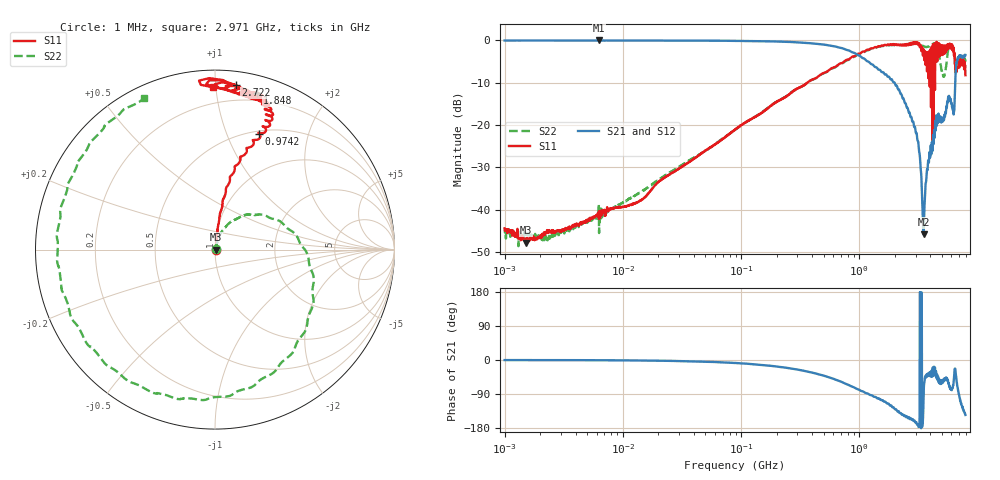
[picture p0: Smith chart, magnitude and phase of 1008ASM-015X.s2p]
!s-Parameter Generated by FASTRON Sdn. Bhd.
!FASTRON P/N : 1008ASM-015X
!Keysight Technologies: E5071C_MY46733604_B.14.02
!Date: Tue Nov 21 10:59:28 2023
!Version  :Rev00  Wed Nov 22 15:44:30 2023
!Data & Calibration Information:
!Freq  S11:SOLT2(ON)  S21:SOLT2(ON)  S12:SOLT2(ON)  S22:SOLT2(ON)
!PortZ  Port1:50+j0  Port2:50+j0
!When reading reference impedance value at option line is always used.
! Remarks : This data is being provided solely for informational purposes.
# Hz S dB R 50
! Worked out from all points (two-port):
!   1599 points, 1 MHz to 7.923 GHz, reference 50 ohm
!   highest |S21| = -0.03 dB at 6.301 MHz (marker M1); lowest = -45.8 dB at 3.508 GHz (marker M2)
!   |S21| within 3 dB of the highest: start of sweep to 920.1 MHz
!   lowest |S11| = -47.8 dB at 1.505 MHz (marker M3), VSWR 1.01, Z = 50.4 + j0.037 ohm
!   |S11| at or under -10 dB: start of sweep to 362.2 MHz; 3.950236 GHz to 3.957143 GHz (6.906 MHz wide, 0.175 % of centre); 4.141 GHz to 4.177 GHz (36.33 MHz wide, 0.873 % of centre)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
!   |S22| runs from -48.6 to -0.6 dB; largest |S21 - S12| = 0.012
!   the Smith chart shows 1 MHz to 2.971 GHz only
!   S11 on the Smith chart (normalised r, x): 1 MHz: 1.01, +0.00; 974.2 MHz: 0.53, +1.31; 1.848 GHz: 0.14, +1.29; 2.722 GHz: 0.09, +1.13; 2.971 GHz: 0.10, +0.98
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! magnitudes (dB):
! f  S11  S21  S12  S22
! 1 MHz  -44.4  0.0  0.0  -44.6
! 1.505 MHz  -47.8  0.0  0.0  -46.2
! 4.479 MHz  -42.9  0.0  -0.1  -43.5
! 6.301 MHz  -40.3  0.0  -0.1  -45.5
! 19.95 MHz  -33.4  -0.1  -0.1  -32.9
! 89.01 MHz  -21.1  -0.1  -0.1  -21.1
! 398.5 MHz  -9.3  -0.7  -0.7  -9.3
! 974.2 MHz  -3.2  -3.5  -3.5  -3.4
! 1.784 GHz  -1.1  -8.6  -8.6  -1.2
! 1.848 GHz  -0.9  -9.2  -9.2  -1.1
! 2.722 GHz  -0.7  -18.1  -18.1  -0.8
! 2.971 GHz  -0.9  -20.5  -20.5  -0.6
! 3.203 GHz  -0.8  -25.9  -25.9  -0.8
! 3.508 GHz  -2.1  -45.8  -45.9  -1.4
! 3.812 GHz  -2.8  -29.6  -29.6  -1.5
! 4.197 GHz  -3.8  -24.3  -24.3  -0.9
! 4.493 GHz  -3.5  -17.7  -17.7  -1.1
! 5.164 GHz  -3.1  -18.2  -18.2  -8.6
! 5.918 GHz  -0.9  -14.4  -14.4  -0.9
! 6.265 GHz  -2.7  -16.7  -16.6  -2.0
! 6.882 GHz  -4.6  -4.3  -4.3  -5.4
! 7.923 GHz  -8.2  -3.4  -3.4  -5.8
